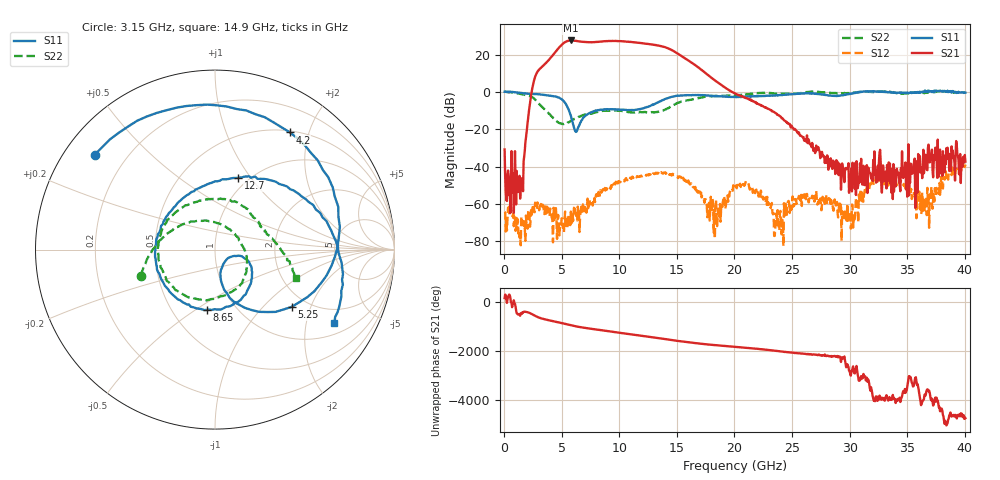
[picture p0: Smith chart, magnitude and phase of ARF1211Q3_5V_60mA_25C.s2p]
!Bias:, VDD=5V, IDD=60mA
# GHz S DB R 50.0
!freq dBS11 angS11 dBS21 angS21 dBS12 angS12 dBS22 angS22
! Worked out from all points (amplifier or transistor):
!   801 points, 50 MHz to 40.05 GHz, reference 50 ohm
!   highest |S21| = 27.5 dB at 5.8 GHz (marker M1)
!   |S21| within 3 dB of that: 4.893 GHz to 13.6 GHz (8.708 GHz wide, 94.2 % of centre)
!   unconditionally stable (mu >= 1): 732.5 MHz to 26.52 GHz; 27.32 GHz to 30.88 GHz; 33.51 GHz to 36.05 GHz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
!   at 6.7 GHz: K = 24.63, MAG = 27.3 dB, |S12| = -61.5 dB
!   at 20.05 GHz: K = 33.39, MAG = 7.2 dB, |S12| = -51.8 dB
!   at 40.05 GHz: K = 20.60, MAG = -15.4 dB, |S12| = -38.9 dB
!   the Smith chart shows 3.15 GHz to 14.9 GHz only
!   S11 on the Smith chart (normalised r, x): 3.15 GHz: 0.09, +0.35; 4.2 GHz: 0.52, +1.71; 5.25 GHz: 1.66, -1.48; 8.65 GHz: 0.73, -0.55; 12.7 GHz: 0.90, +0.87; 14.9 GHz: 1.40, -2.93
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0.05  0.09 -2.6  -30.79 158.5  -64.14 13.6  0.03 -1.7
3.15  -1.38 141.7  12.59 66.7  -60.70 86.0  -7.18 -160.6
4.2  -2.22 57.4  19.38 -53.5  -68.80 45.6  -13.57 134.1
4.8  -3.18 5.7  23.90 -115.0  -76.76 98.2  -16.65 81.9
5.25  -5.47 -36.8  26.48 -166.3  -68.66 16.3  -17.00 38.5
5.8  -12.78 -77.2  27.52 131.7  -64.07 159.8  -15.45 -3.9
6.2  -21.10 -52.6  27.33 92.6  -64.65 139.9  -14.22 -24.2
6.75  -15.16 -16.9  26.83 47.0  -64.23 123.8  -12.75 -47.1
7.65  -10.72 -52.1  26.56 -15.4  -59.64 129.9  -11.50 -85.4
8.65  -9.41 -98.0  27.05 -80.3  -52.84 116.2  -10.13 -132.5
9.35  -9.26 -132.0  27.21 -127.1  -51.69 103.8  -9.96 -167.5
10.25  -9.50 -175.8  27.06 173.3  -47.22 71.6  -10.24 145.4
11.45  -9.54 127.8  26.47 96.9  -45.12 32.7  -10.92 81.9
12.7  -7.51 71.9  25.46 18.8  -44.28 -16.0  -10.97 36.9
13.4  -5.45 41.2  24.81 -26.8  -43.56 -43.1  -10.51 21.2
14.1  -3.54 6.4  23.64 -75.9  -43.61 -74.2  -9.07 3.8
14.9  -2.16 -31.5  21.22 -131.5  -44.77 -110.1  -6.42 -19.2
16.55  -1.75 -91.0  14.52 132.1  -51.63 -169.4  -3.80 -65.2
20.05  -2.66 -169.0  -0.79 -22.2  -51.76 -102.8  -1.79 -146.2
26.75  -0.90 103.9  -27.30 11.6  -55.59 36.6  0.00 117.4
33.4  -0.28 37.7  -37.70 3.5  -48.21 2.8  0.11 43.8
40.05  -0.41 -54.5  -37.33 -44.6  -38.87 18.8  -0.33 -39.5
